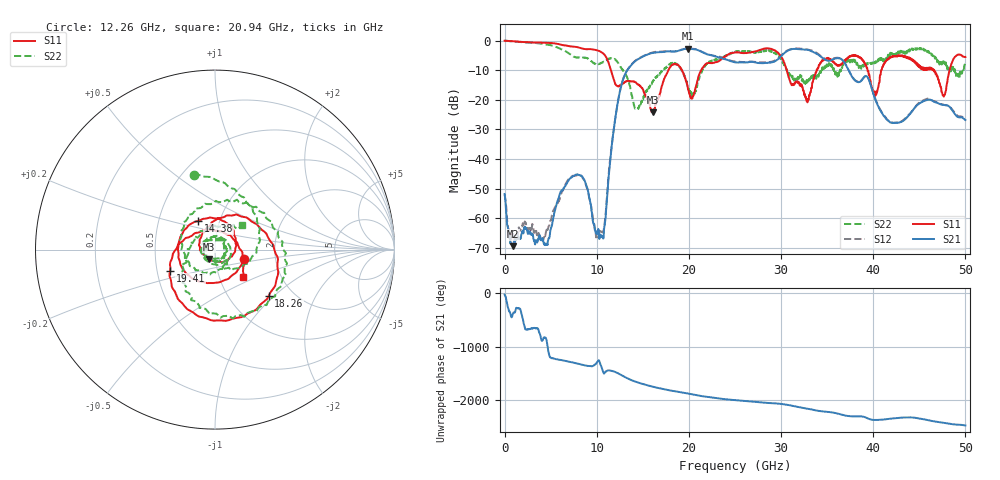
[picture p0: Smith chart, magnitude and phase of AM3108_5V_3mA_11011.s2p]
# Hz S DB R 50.0
!freq dBS11 angS11 dBS21 angS21 dBS12 angS12 dBS22 angS22
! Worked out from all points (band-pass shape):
!   1601 points, 10 MHz to 50 GHz, reference 50 ohm
!   highest |S21| = -2.71 dB at 19.91 GHz (marker M1); lowest = -69.4 dB at 916.1 MHz (marker M2)
!   |S21| within 3 dB of the highest: 14.82 GHz to 23.33 GHz (8.511 GHz wide, 44.6 % of centre); 29.87 GHz to 34.45 GHz (4.578 GHz wide, 14.2 % of centre)
!   lowest |S11| = -24.2 dB at 16.07 GHz (marker M3), VSWR 1.13, Z = 46.6 - j4.94 ohm
!   |S11| at or under -10 dB: 11.55 GHz to 17.78 GHz (6.228 GHz wide, 42.5 % of centre); 19.26 GHz to 21.34 GHz (2.079 GHz wide, 10.2 % of centre); 30.63 GHz to 33.85 GHz (3.225 GHz wide, 10 % of centre)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
!   |S22| runs from -23.2 to 0.1 dB; largest |S21 - S12| = 0.028
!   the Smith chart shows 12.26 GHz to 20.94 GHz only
!   S11 on the Smith chart (normalised r, x): 12.26 GHz: 1.38, -0.14; 14.38 GHz: 0.79, +0.26; 18.26 GHz: 1.51, -0.93; 19.41 GHz: 0.59, -0.15; 20.94 GHz: 1.29, -0.41
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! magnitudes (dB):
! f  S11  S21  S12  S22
! 10 MHz  0.0  -51.8  -51.9  0.1
! 916.1 MHz  -0.2  -69.4  -65.3  -0.3
! 4.509 GHz  -0.7  -68.7  -64.4  -1.3
! 6.165 GHz  -1.4  -50.7  -51.6  -2.9
! 8.352 GHz  -2.6  -45.8  -45.6  -5.7
! 10.54 GHz  -3.9  -65.9  -64.7  -7.5
! 12.26 GHz  -15.4  -21.4  -21.4  -7.3
! 14.38 GHz  -14.6  -6.5  -6.3  -23.0
! 16.07 GHz  -24.2  -4.2  -4.0  -13.9
! 16.69 GHz  -19.3  -3.9  -3.7  -11.9
! 18.26 GHz  -8.0  -3.7  -3.6  -7.7
! 19.41 GHz  -11.2  -2.9  -2.8  -11.0
! 19.91 GHz  -16.5  -2.7  -2.6  -15.6
! 20.94 GHz  -13.3  -3.2  -3.0  -13.9
! 25 GHz  -4.0  -7.3  -7.0  -3.9
! 29.13 GHz  -3.0  -7.2  -7.0  -3.8
! 33.35 GHz  -15.7  -3.6  -3.3  -12.7
! 38 GHz  -4.9  -13.4  -13.3  -6.5
! 40.22 GHz  -18.7  -19.8  -19.6  -7.6
! 41.69 GHz  -6.0  -27.2  -27.1  -5.2
! 47.66 GHz  -18.9  -21.7  -21.7  -7.7
! 50 GHz  -5.5  -26.8  -26.6  -6.9
